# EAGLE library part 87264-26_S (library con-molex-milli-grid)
RECEPTACAL
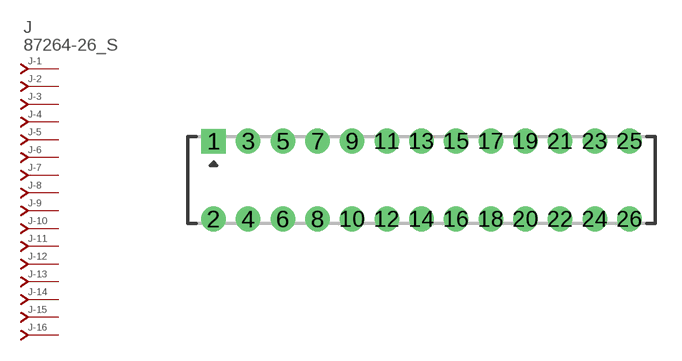
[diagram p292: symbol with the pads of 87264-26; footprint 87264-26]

Designator prefix J; gates -1=J-NV -2=J-N -3=J-N -4=J-N -5=J-N -6=J-N -7=J-N -8=J-N -9=J-N -10=J-N -11=J-N -12=J-N -13=J-N -14=J-N -15=J-N -16=J-N -17=J-N -18=J-N -19=J-N -20=J-N -21=J-N -22=J-N -23=J-N -24=J-N -25=J-N -26=J-N

## 87264-26_S  [87264-26]
1  -1:J  pas
2  -2:J  pas
3  -3:J  pas
4  -4:J  pas
5  -5:J  pas
6  -6:J  pas
7  -7:J  pas
8  -8:J  pas
9  -9:J  pas
10  -10:J  pas
11  -11:J  pas
12  -12:J  pas
13  -13:J  pas
14  -14:J  pas
15  -15:J  pas
16  -16:J  pas
17  -17:J  pas
18  -18:J  pas
19  -19:J  pas
20  -20:J  pas
21  -21:J  pas
22  -22:J  pas
23  -23:J  pas
24  -24:J  pas
25  -25:J  pas
26  -26:J  pas

## Footprint 87264-26 (pad centres in mm)
RECEPTACAL Dual Row, Side Entry
drill 0.914 square: 1 -12,2.25
drill 0.914: 2 -12,-2.25; 3 -10,2.25; 4 -10,-2.25; 5 -8,2.25; 6 -8,-2.25; 7 -6,2.25; 8 -6,-2.25; 9 -4,2.25; 10 -4,-2.25; 11 -2,2.25; 12 -2,-2.25; 13 0,2.25; 14 0,-2.25; 15 2,2.25; 16 2,-2.25; 17 4,2.25; 18 4,-2.25; 19 6,2.25; 20 6,-2.25; 21 8,2.25; 22 8,-2.25; 23 10,2.25; 24 10,-2.25; 25 12,2.25; 26 12,-2.25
